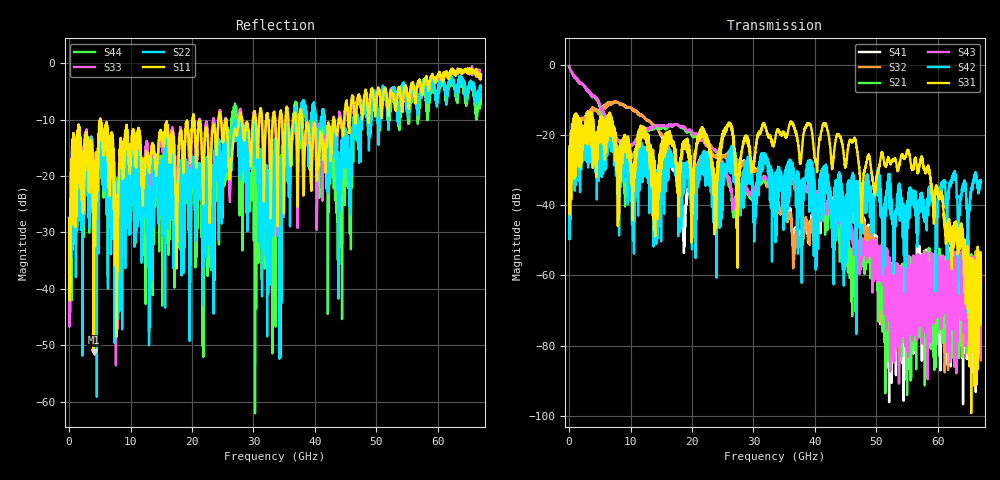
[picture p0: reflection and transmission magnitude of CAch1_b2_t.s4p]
!Agilent Technologies,N5247A,US51170199,A.09.90.13
!Agilent N5247A: A.09.90.13
!Date: Tuesday, October 23, 2018 11:12:37
!Correction: S11(Full 4 Port(1,2,3,4))
!S12(Full 4 Port(1,2,3,4))
!S13(Full 4 Port(1,2,3,4))
!S14(Full 4 Port(1,2,3,4))
!S21(Full 4 Port(1,2,3,4))
!S22(Full 4 Port(1,2,3,4))
!S23(Full 4 Port(1,2,3,4))
!S24(Full 4 Port(1,2,3,4))
!S31(Full 4 Port(1,2,3,4))
!S32(Full 4 Port(1,2,3,4))
!S33(Full 4 Port(1,2,3,4))
!S34(Full 4 Port(1,2,3,4))
!S41(Full 4 Port(1,2,3,4))
!S42(Full 4 Port(1,2,3,4))
!S43(Full 4 Port(1,2,3,4))
!S44(Full 4 Port(1,2,3,4))
!S4P File: Measurements: <S11,S12,S13,S14>,
!<S21,S22,S23,S24>,
!<S31,S32,S33,S34>,
!<S41,S42,S43,S44>:
# Hz S  dB  R 50
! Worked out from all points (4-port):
!   6701 points, 10 MHz to 67 GHz, reference 50 ohm
!   strongest paths, dB at 10 MHz, 16.76 GHz, 33.51 GHz, 50.25 GHz, 67 GHz:
!     S31: -32.8, -22.9, -21.4, -30.3, -57.7
!     S42: -33.1, -25.6, -31.6, -36.2, -33.0
!     S43: -0.4, -17.3, -31.6, -55.4, -59.5
!     S21: -0.4, -17.3, -32.4, -55.2, -60.6
!     S32: -46.7, -26.4, -37.9, -53.4, -60.2
!     S41: -46.9, -28.3, -37.5, -59.5, -60.0
!   lowest |S11| = -51.3 dB at 3.989 GHz (marker M1), VSWR 1.01, Z = 50.3 - j0.082 ohm
!   |S11| at or under -10 dB: start of sweep to 5.069 GHz; 5.093 GHz to 20.11 GHz (15.02 GHz wide, 119 % of centre); 37.88 GHz to 43.05 GHz (5.166 GHz wide, 12.8 % of centre)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
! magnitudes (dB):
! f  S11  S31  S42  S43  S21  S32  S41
! 10 MHz  -27.5  -32.8  -33.1  -0.4  -0.4  -46.7  -46.9
! 3.989 GHz  -51.3  -25.1  -27.7  -8.8  -8.9  -12.4  -12.4
! 9.139 GHz  -15.2  -22.6  -26.3  -22.9  -34.2  -11.8  -11.7
! 17.56 GHz  -30.4  -33.6  -32.7  -17.0  -17.0  -29.0  -31.4
! 44.48 GHz  -11.4  -22.6  -36.7  -43.1  -46.7  -39.7  -39.5
! 55.12 GHz  -6.5  -24.3  -46.1  -72.2  -64.5  -60.2  -58.8
! 67 GHz  -2.0  -57.7  -33.0  -59.5  -60.6  -60.2  -60.0
